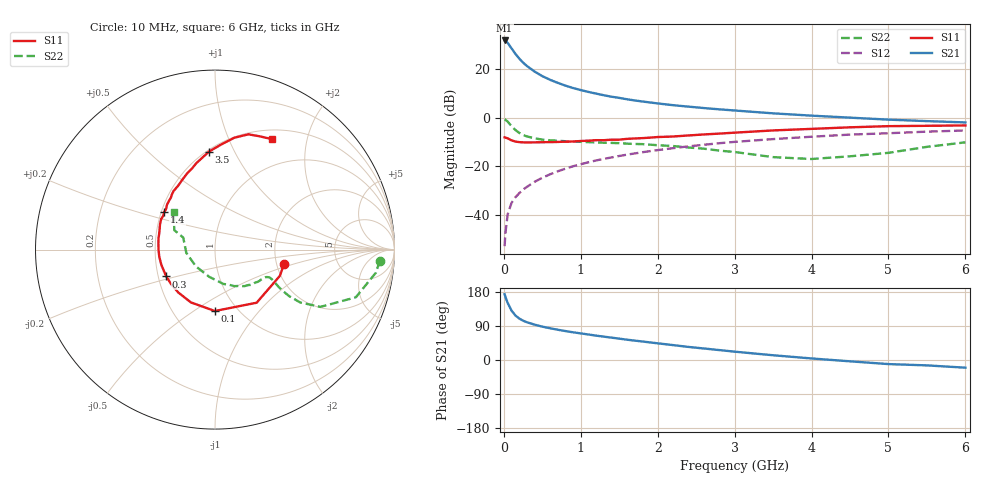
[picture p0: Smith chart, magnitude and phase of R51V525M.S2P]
! SIEMENS Small Signal Semiconductors
! BFR183
! Si NPN RF Bipolar Junction Transistor in SOT23
! VCE = 1.5 V  IC = 25 mA
! Common Emitter S-Parameters:  May  1996
# GHz  S  MA  R  50
!  f  S11  S21  S12  S22
! GHz  MAG  ANG  MAG  ANG  MAG  ANG  MAG  ANG
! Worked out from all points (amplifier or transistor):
!   36 points, 10 MHz to 6 GHz, reference 50 ohm
!   highest |S21| = 31.7 dB at 10 MHz (marker M1)
!   |S21| within 3 dB of that: start of sweep to 94.55 MHz
!   unconditionally stable (mu >= 1): 385.8 MHz to 2.529 GHz
!   at 250 MHz: K = 0.90, MSG = 26.1 dB, |S12| = -29.5 dB
!   at 1.4 GHz: K = 1.07, MAG = 10.8 dB, |S12| = -16.3 dB
!   at 6 GHz: K = 0.94, MSG = 1.7 dB, |S12| = -5.3 dB
!   S11 on the Smith chart (normalised r, x): 10 MHz: 2.20, -0.41; 100 MHz: 0.79, -0.61; 300 MHz: 0.55, -0.18; 1.4 GHz: 0.52, +0.25; 3.5 GHz: 0.51, +0.80; 6 GHz: 0.62, +1.46
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0.01  0.3934 -11.4  38.42 173.5  0.0023 88.7  0.9201 -3.8
0.02  0.39 -22.0  37.89 167.0  0.0042 80.3  0.9061 -8.1
0.05  0.3761 -51.9  34.29 150.3  0.0104 74.7  0.8286 -18.7
0.1  0.3421 -90.2  26.44 130.3  0.0178 69.6  0.6688 -28.5
0.15  0.3234 -114.5  20.44 117.6  0.0232 66.0  0.5588 -31.8
0.2  0.3146 -130.7  16.37 109.5  0.0281 67.9  0.4869 -32.1
0.25  0.3108 -142.5  13.5 103.8  0.0334 68.5  0.4399 -31.3
0.3  0.3101 -151.1  11.5 99.6  0.0379 70.0  0.4115 -30.4
0.4  0.3108 -164.0  8.829 93.3  0.0482 70.9  0.3761 -28.6
0.5  0.3131 -172.9  7.113 88.0  0.0583 71.8  0.3544 -27.4
0.6  0.3146 -179.7  5.993 83.8  0.0686 71.8  0.343 -27.1
0.7  0.3173 173.9  5.184 79.9  0.079 71.7  0.3356 -27.3
0.8  0.321 168.7  4.546 76.4  0.0896 71.2  0.3283 -27.8
0.9  0.3238 163.5  4.057 73.1  0.1005 70.6  0.3228 -28.3
1.1  0.3372 155.4  3.37 67.3  0.1213 69.4  0.314 -30.9
1.4  0.3528 143.3  2.689 59.0  0.1526 66.3  0.3031 -35.0
1.7  0.3734 133.4  2.255 51.2  0.1841 63.0  0.2885 -40.2
2.2  0.4102 120.2  1.802 39.3  0.2364 57.1  0.2614 -51.2
3.5  0.5465 93.6  1.226 12.5  0.3628 39.3  0.1547 -102.3
4.5  0.6331 80.1  1 -3.5  0.4488 25.8  0.1609 -173.5
5.5  0.68 67.8  0.849 -14.2  0.516 13.7  0.2514 154.5
6  0.6924 62.6  0.798 -20.3  0.5456 6.0  0.3114 137.5
